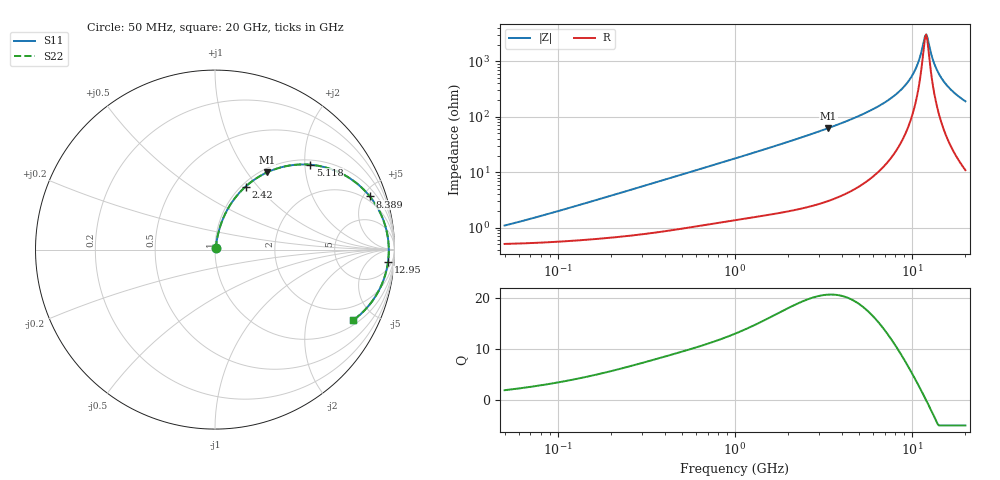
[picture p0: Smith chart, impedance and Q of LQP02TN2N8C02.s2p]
!Murata Part Number: LQP02TN2N8C02
!These Parameters are Measured in Series Mode Connection
!  o--[Z]--o
!Port1  Port2
!  o-------o
!Freq. Start=50[MHz] Stop=20[GHz], 401[Steps]
# Hz S RI R 50
!Freq.(Hz) S11(Real) S11(Imag) S21(Real) S21(Imag) S12(Real) S12(Imag) S22(Real) S22(Imag)
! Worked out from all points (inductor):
!   401 points, 50 MHz to 20 GHz, reference 50 ohm
!   read as one part in series: L = 3.03 nH near 85.73 MHz
!   highest Q = 20.6 at 3.364 GHz (marker M1), where L = 2.95 nH
!   self-resonance near 11.84 GHz
!   S11 on the Smith chart (normalised r, x): 50 MHz: 1.01, +0.02; 2.42 GHz: 1.04, +0.87; 5.118 GHz: 1.11, +2.13; 8.389 GHz: 1.57, +5.56; 12.95 GHz: 10, -22; 20 GHz: 1.22, -3.81
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5e7  0.00516 0.00958  0.9948 -0.00958  0.9948 -0.00958  0.00516 0.00958
1.364002e8  0.00658 0.0254  0.9934 -0.0254  0.9934 -0.0254  0.00658 0.0254
3.721004e8  0.0127 0.0665  0.9873 -0.0665  0.9873 -0.0665  0.0127 0.0665
1e9  0.0426 0.1669  0.9574 -0.1669  0.9574 -0.1669  0.0426 0.1669
1.639343e9  0.0906 0.2582  0.9094 -0.2582  0.9094 -0.2582  0.0906 0.2582
2.419936e9  0.1707 0.3513  0.8293 -0.3513  0.8293 -0.3513  0.1707 0.3513
2.728004e9  0.2076 0.3813  0.7924 -0.3813  0.7924 -0.3813  0.2076 0.3813
3.364474e9  0.2902 0.4303  0.7098 -0.4303  0.7098 -0.4303  0.2902 0.4303
5.117541e9  0.5313 0.4728  0.4687 -0.4728  0.4687 -0.4728  0.5313 0.4728
7.442007e9  0.7911 0.3682  0.2089 -0.3682  0.2089 -0.3682  0.7911 0.3682
8.389408e9  0.8627 0.2963  0.1373 -0.2963  0.1373 -0.2963  0.8627 0.2963
9.457416e9  0.9193 0.2076  0.0807 -0.2076  0.0807 -0.2076  0.9193 0.2076
1.034674e10  0.9487 0.1323  0.0513 -0.1323  0.0513 -0.1323  0.9487 0.1323
1.098561e10  0.9612 0.0792  0.0388 -0.0792  0.0388 -0.0792  0.9612 0.0792
1.166392e10  0.9676 0.0248  0.0324 -0.0248  0.0324 -0.0248  0.9676 0.0248
1.183995e10  0.9682 0.0111  0.0318 -0.0111  0.0318 -0.0111  0.9682 0.0111
1.220001e10  0.9683 -0.0164  0.0317 0.0164  0.0317 0.0164  0.9683 -0.0164
1.295331e10  0.9637 -0.0712  0.0363 0.0712  0.0363 0.0712  0.9637 -0.0712
1.396067e10  0.9493 -0.1381  0.0507 0.1381  0.0507 0.1381  0.9493 -0.1381
1.527346e10  0.9201 -0.2139  0.0799 0.2139  0.0799 0.2139  0.9201 -0.2139
1.721783e10  0.8635 -0.3037  0.1365 0.3037  0.1365 0.3037  0.8635 -0.3037
2e10  0.7716 -0.3921  0.2284 0.3921  0.2284 0.3921  0.7716 -0.3921
